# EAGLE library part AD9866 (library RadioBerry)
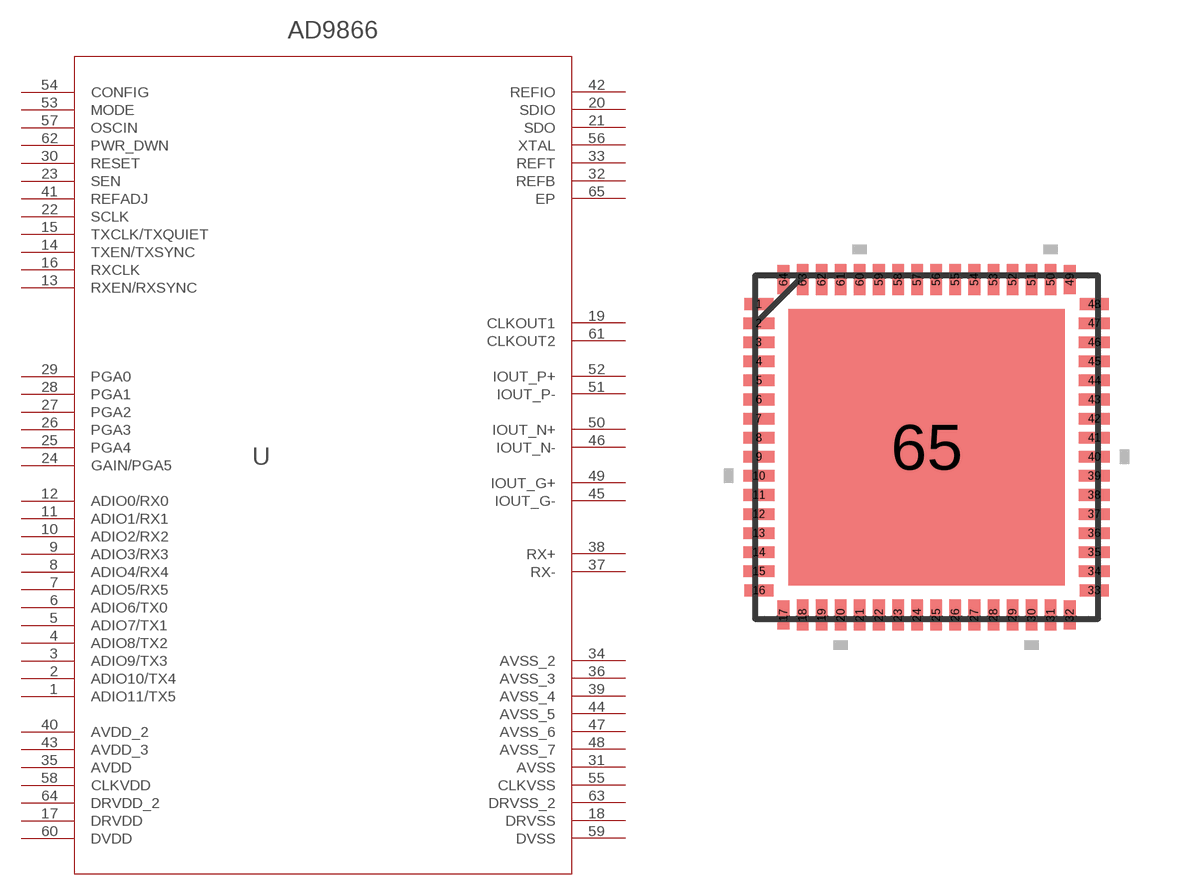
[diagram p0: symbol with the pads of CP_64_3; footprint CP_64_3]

Designator prefix -

## AD9866  [CP_64_3]
1  ADIO11/TX5  pas
2  ADIO10/TX4  pas
3  ADIO9/TX3  pas
4  ADIO8/TX2  pas
5  ADIO7/TX1  pas
6  ADIO6/TX0  pas
7  ADIO5/RX5  pas
8  ADIO4/RX4  pas
9  ADIO3/RX3  pas
10  ADIO2/RX2  pas
11  ADIO1/RX1  pas
12  ADIO0/RX0  pas
13  RXEN/RXSYNC  pas
14  TXEN/TXSYNC  pas
15  TXCLK/TXQUIET  pas
16  RXCLK  pas
17  DRVDD  pwr
18  DRVSS  pas
19  CLKOUT1  pas
20  SDIO  pas
21  SDO  pas
22  SCLK  pas
23  SEN  pas
24  GAIN/PGA5  pas
25  PGA4  pas
26  PGA3  pas
27  PGA2  pas
28  PGA1  pas
29  PGA0  pas
30  RESET  pas
31  AVSS  pas
32  REFB  pas
33  REFT  pas
34  AVSS_2  pas
35  AVDD  pwr
36  AVSS_3  pas
37  RX-  pas
38  RX+  pas
39  AVSS_4  pas
40  AVDD_2  pwr
41  REFADJ  pas
42  REFIO  pas
43  AVDD_3  pwr
44  AVSS_5  pas
45  IOUT_G-  pas
46  IOUT_N-  pas
47  AVSS_6  pas
48  AVSS_7  pas
49  IOUT_G+  pas
50  IOUT_N+  pas
51  IOUT_P-  pas
52  IOUT_P+  pas
53  MODE  pas
54  CONFIG  pas
55  CLKVSS  pas
56  XTAL  pas
57  OSCIN  pas
58  CLKVDD  pwr
59  DVSS  pas
60  DVDD  pwr
61  CLKOUT2  pas
62  PWR_DWN  pas
63  DRVSS_2  pas
64  DRVDD_2  pwr
65  EP  pas

## Footprint CP_64_3 (pad centres in mm)
smd 0.762 x 0.305: 1 -4.394,3.75; 16 -4.394,-3.75; 33 4.394,-3.75; 48 4.394,3.75
smd 0.813 x 0.305: 2 -4.394,3.25; 3 -4.394,2.75; 4 -4.394,2.25; 5 -4.394,1.75; 6 -4.394,1.25; 7 -4.394,0.75; 8 -4.394,0.25; 9 -4.394,-0.25; 10 -4.394,-0.75; 11 -4.394,-1.25; 12 -4.394,-1.75; 13 -4.394,-2.25; 14 -4.394,-2.75; 15 -4.394,-3.25; 34 4.394,-3.25; 35 4.394,-2.75; 36 4.394,-2.25; 37 4.394,-1.75; 38 4.394,-1.25; 39 4.394,-0.75; 40 4.394,-0.25; 41 4.394,0.25; 42 4.394,0.75; 43 4.394,1.25; 44 4.394,1.75; 45 4.394,2.25; 46 4.394,2.75; 47 4.394,3.25
smd 0.305 x 0.762: 17 -3.75,-4.394; 32 3.75,-4.394; 49 3.75,4.394; 64 -3.75,4.394
smd 0.305 x 0.813: 18 -3.25,-4.394; 19 -2.75,-4.394; 20 -2.25,-4.394; 21 -1.75,-4.394; 22 -1.25,-4.394; 23 -0.75,-4.394; 24 -0.25,-4.394; 25 0.25,-4.394; 26 0.75,-4.394; 27 1.25,-4.394; 28 1.75,-4.394; 29 2.25,-4.394; 30 2.75,-4.394; 31 3.25,-4.394; 50 3.25,4.394; 51 2.75,4.394; 52 2.25,4.394; 53 1.75,4.394; 54 1.25,4.394; 55 0.75,4.394; 56 0.25,4.394; 57 -0.25,4.394; 58 -0.75,4.394; 59 -1.25,4.394; 60 -1.75,4.394; 61 -2.25,4.394; 62 -2.75,4.394; 63 -3.25,4.394
smd 7.239 x 7.239: 65 0,0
